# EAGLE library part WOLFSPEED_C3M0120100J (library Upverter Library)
Silicon Carbide Power MOSFET N-Channel 1000 V 22A (Tc) 83W (Tc) RDS(on) 120mohm
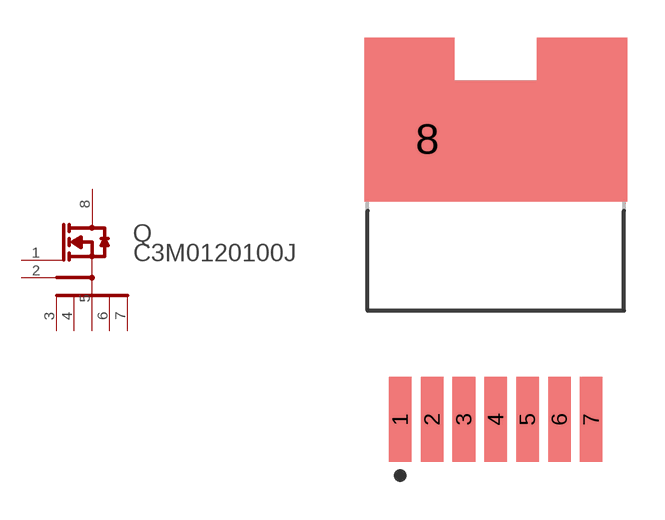
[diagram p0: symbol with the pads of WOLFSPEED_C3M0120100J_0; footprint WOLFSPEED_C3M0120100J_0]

Designator prefix Q

## WOLFSPEED_C3M0120100JWOLFSPEED_C3M0120100J_0_0 (MF: Wolfspeed; MPN: C3M0120100J; automotive: No; centroid_not_specified: Yes; continuous_drain_current: 22A; datasheet: https://assets.wolfspeed.com/uploads/2020/12/c3m0120100j.pdf; depletion_mode: False; device_class_L1: Discrete Semiconductors; device_class_L2: Transistors; device_class_L3: MOSFETs; digikey_description: SICFET N-CH 1000V 22A D2PAK-7; digikey_part_number: C3M0120100J-ND; drain_to_source_breakdown_voltage: 1000V; drain_to_source_resistance: 120mΩ; drain_to_source_voltage: 1000V; footprint_variant_name_0: Recommended_Land_Pattern; gate_charge_at_vgs: 18nC @ 15V; gate_to_source_voltage: 19V; height: 4.82mm; input_capacitace_at_vds: 414pF @ 600V; lead_free: Yes; max_junction_temp: +150°C; mfg_package_ident: TO-263-7; mfg_package_ident_component_id: d2de6d38281de76c; mfg_package_ident_date: 0; mfg_package_ident_rev: 0; mouser_part_number: 941-C3M0120100J; number_of_N_channels: 1; number_of_channels: 1; package: TO-263-7; power_dissipation: 83W; prefix: Q; pulse_drain_current: 50A; reverse_recovery_charge: 78nC; reverse_recovery_time: 10ns; rohs: Yes; rthja_max: 40°C/W; standoff_height: 0mm; technology: SiC; temperature_range_high: +150°C; temperature_range_low: -55°C; threshold_vgs_max: 3.5V; threshold_vgs_min: 1.8V; transconductance: 8.9S; turn_off_delay_time: 14ns; turn_on_delay_time: 6ns; typ_forward_diode_voltage: 4.8V; verification_version: 0.0.0.3)  [WOLFSPEED_C3M0120100J_0]
1  GATE  pas
2  DRIVER_SOURCE  pas
3  1_POWER_SOURCE  pas
4  2_POWER_SOURCE  pas
5  3_POWER_SOURCE  pas
6  4_POWER_SOURCE  pas
7  5_POWER_SOURCE  pas
8  DRAIN  pas

## Footprint WOLFSPEED_C3M0120100J_0 (pad centres in mm)
Silicon Carbide Power MOSFET N-Channel 1000 V 22A (Tc) 83W (Tc) RDS(on) 120mohm
smd 0.9 x 3.4: 1 -3.81,-6.764; 2 -2.54,-6.764; 3 -1.27,-6.764; 4 0,-6.764; 5 1.27,-6.764; 6 2.54,-6.764; 7 3.81,-6.764
smd 4.505 x 4.505: 8 -2.737,4.429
